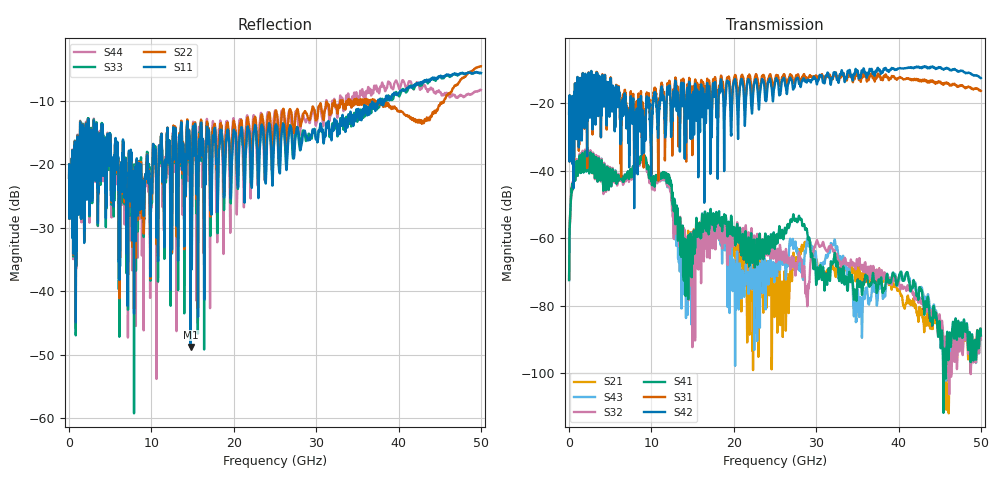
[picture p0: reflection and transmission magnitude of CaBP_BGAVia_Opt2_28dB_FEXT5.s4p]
!* Samtec Inc. NovaRay Examax Flyover System  *
!*  REV DATE  = 08/08/18  *
!*  TYPE  = TOUCHSTONE  *
!*  PORTS  = 4 port  *
!*  UNITS  = GHz  *
!*  DATA RANGE = DC  to 50 GHz; 10 MHz Step  *
!*  PARAMETER  = S  *
!*  FORMAT  = Real-Imaginary  *
!*  REFERENCE  = 50 ohms  *
!*  SOURCE  = HFSS  *
!*  VALIDATED  = No  *
!*  MANUFACTURER = SAMTEC  *
!*  INTERCONNECT = NVAx to EBCx to EBCx to NVAx  *
!*  [Full Channel NVAx to EBCx to EBCx to NVAx  with PCB Trace and BGA Via]  *
!*  BOUNDARY A  = Silicon BGA Ball Pad  *
!*  BOUNDARY B  = Silicon BGA Ball Pad  *
!*  NVAx (end a) ->>- (end b) NVAx  *
!*  Port 01 ->>- Port 02  *
!*  Port 03 ->>- Port 04  *
!***************************** CHANNEL MODEL ******************************************
# GHz S RI R 50
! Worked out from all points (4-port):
!   5000 points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, 10 MHz to 50 GHz, reference 50 ohm
!   strongest paths, dB at 10 MHz, 12.51 GHz, 25.01 GHz, 37.51 GHz, 50 GHz:
!     S42: -23.1, -24.5, -14.1, -9.6, -12.6
!     S31: -23.1, -28.5, -13.0, -11.3, -16.4
!     S41: -72.4, -47.9, -62.4, -74.4, -88.8
!     S32: -71.8, -51.7, -64.3, -72.1, -89.9
!     S43: -72.0, -50.6, -69.8, -76.2, -90.0
!     S21: -72.1, -49.4, -74.6, -72.4, -88.8
!   lowest |S11| = -48.8 dB at 14.75 GHz (marker M1), VSWR 1.01, Z = 49.7 - j0.221 ohm
!   |S11| at or under -10 dB: start of sweep to 37.51 GHz; 37.83997 GHz to 38.00552 GHz (165.6 MHz wide, 0.437 % of centre); 38.04261 GHz to 38.22467 GHz (182.1 MHz wide, 0.477 % of centre)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
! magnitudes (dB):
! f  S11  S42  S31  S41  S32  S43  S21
! 10 MHz  -22.1  -23.1  -23.1  -72.4  -71.8  -72.0  -72.1
! 1.1 GHz  -17.2  -15.0  -15.2  -40.0  -39.6  -39.7  -39.8
! 9.02 GHz  -25.1  -26.1  -24.5  -35.5  -36.1  -35.8  -35.6
! 14.75 GHz  -48.8  -28.6  -22.0  -59.5  -60.6  -64.8  -60.2
! 16.36 GHz  -22.5  -20.6  -17.2  -56.5  -66.4  -57.8  -59.8
! 20.76 GHz  -15.5  -15.0  -14.6  -57.4  -56.9  -69.2  -59.7
! 50 GHz  -5.6  -12.6  -16.4  -88.8  -89.9  -90.0  -88.8
